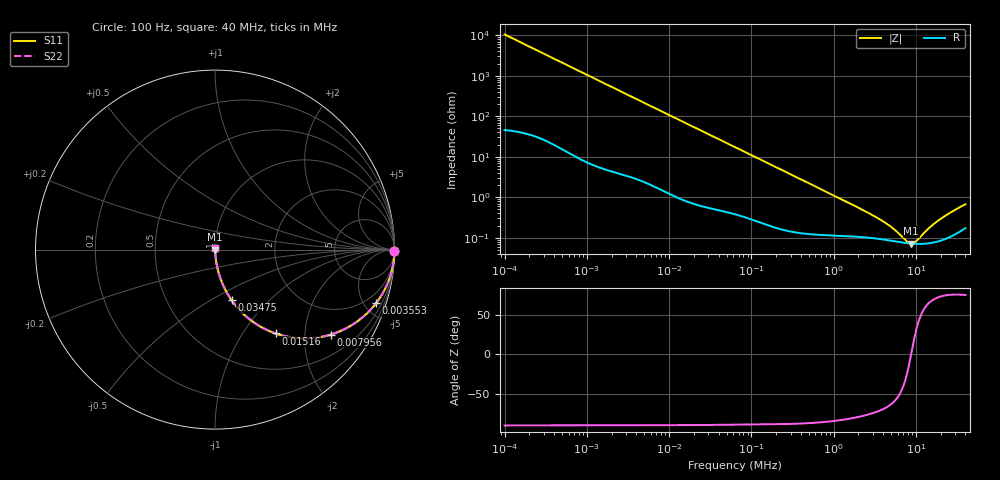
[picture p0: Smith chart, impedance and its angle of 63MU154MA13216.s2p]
!Components F PML CAP
!CONCATENATE F 0.1-40000kHz, at 20deg DC=0V
!Part Number F 63MU154MA13216
!Copyright(C) Rubycon Corporation. 20161129
# MHz S MA R 50
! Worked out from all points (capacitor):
!   561 points, 100 Hz to 40 MHz, reference 50 ohm
!   read as one part in series: C = 152 nF near 104.7 Hz
!   lowest |Z| = 71.9 mohm at 8.746 MHz (marker M1)
!   series resonance near 8.753 MHz, so ESL is about 2.2 nH
!   S11 on the Smith chart (normalised r, x): 100 Hz: open; 3.553 kHz: 1.06, -6.00; 7.956 kHz: 1.03, -2.70; 15.16 kHz: 1.02, -1.42; 34.75 kHz: 1.01, -0.62; 40 MHz: 1.00, +0.01
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0.0001  0.9999 -0.5  0.009536 89.2  0.009536 89.2  0.9999 -0.5
0.0008716573  0.9961 -4.7  0.08193 84.9  0.08193 84.9  0.9961 -4.7
0.001821644  0.9843 -9.7  0.1688 79.8  0.1688 79.8  0.9843 -9.7
0.003552795  0.9458 -18.4  0.3152 71.0  0.3152 71.0  0.9458 -18.4
0.005136048  0.8975 -25.5  0.4311 63.8  0.4311 63.8  0.8975 -25.5
0.007424854  0.8179 -34.5  0.5662 54.9  0.5662 54.9  0.8179 -34.5
0.007956076  0.7989 -36.3  0.5924 53.0  0.5924 53.0  0.7989 -36.3
0.01098374  0.6956 -45.3  0.7106 44.1  0.7106 44.1  0.6956 -45.3
0.01516359  0.5759 -54.2  0.8108 35.2  0.8108 35.2  0.5759 -54.2
0.02295452  0.4233 -64.2  0.9004 25.0  0.9004 25.0  0.4233 -64.2
0.03474836  0.2959 -71.9  0.9504 17.2  0.9504 17.2  0.2959 -71.9
0.06324555  0.1691 -79.0  0.9819 9.7  0.9819 9.7  0.1691 -79.0
0.1589195  0.0691 -84.4  0.9956 4.0  0.9956 4.0  0.0691 -84.4
0.5512845  0.0201 -85.4  0.9986 1.1  0.9986 1.1  0.0201 -85.4
2.580015  0.004215 -75.9  0.999 0.2  0.999 0.2  0.004215 -75.9
4.69589  0.002036 -64.9  0.9991 0.1  0.9991 0.1  0.002036 -64.9
7.794689  0.0008102 -24.7  0.9993 0.0  0.9993 0.0  0.0008102 -24.7
8.746156  0.0007186 -0.2  0.9993 0.0  0.9993 0.0  0.0007186 -0.2
10.04244  0.000816 30.1  0.9993 -0.0  0.9993 -0.0  0.000816 30.1
14.18713  0.001678 64.3  0.9993 -0.1  0.9993 -0.1  0.001678 64.3
19.14002  0.002748 72.4  0.9992 -0.2  0.9992 -0.2  0.002748 72.4
40  0.006719 74.7  0.9982 -0.4  0.9982 -0.4  0.006719 74.7
